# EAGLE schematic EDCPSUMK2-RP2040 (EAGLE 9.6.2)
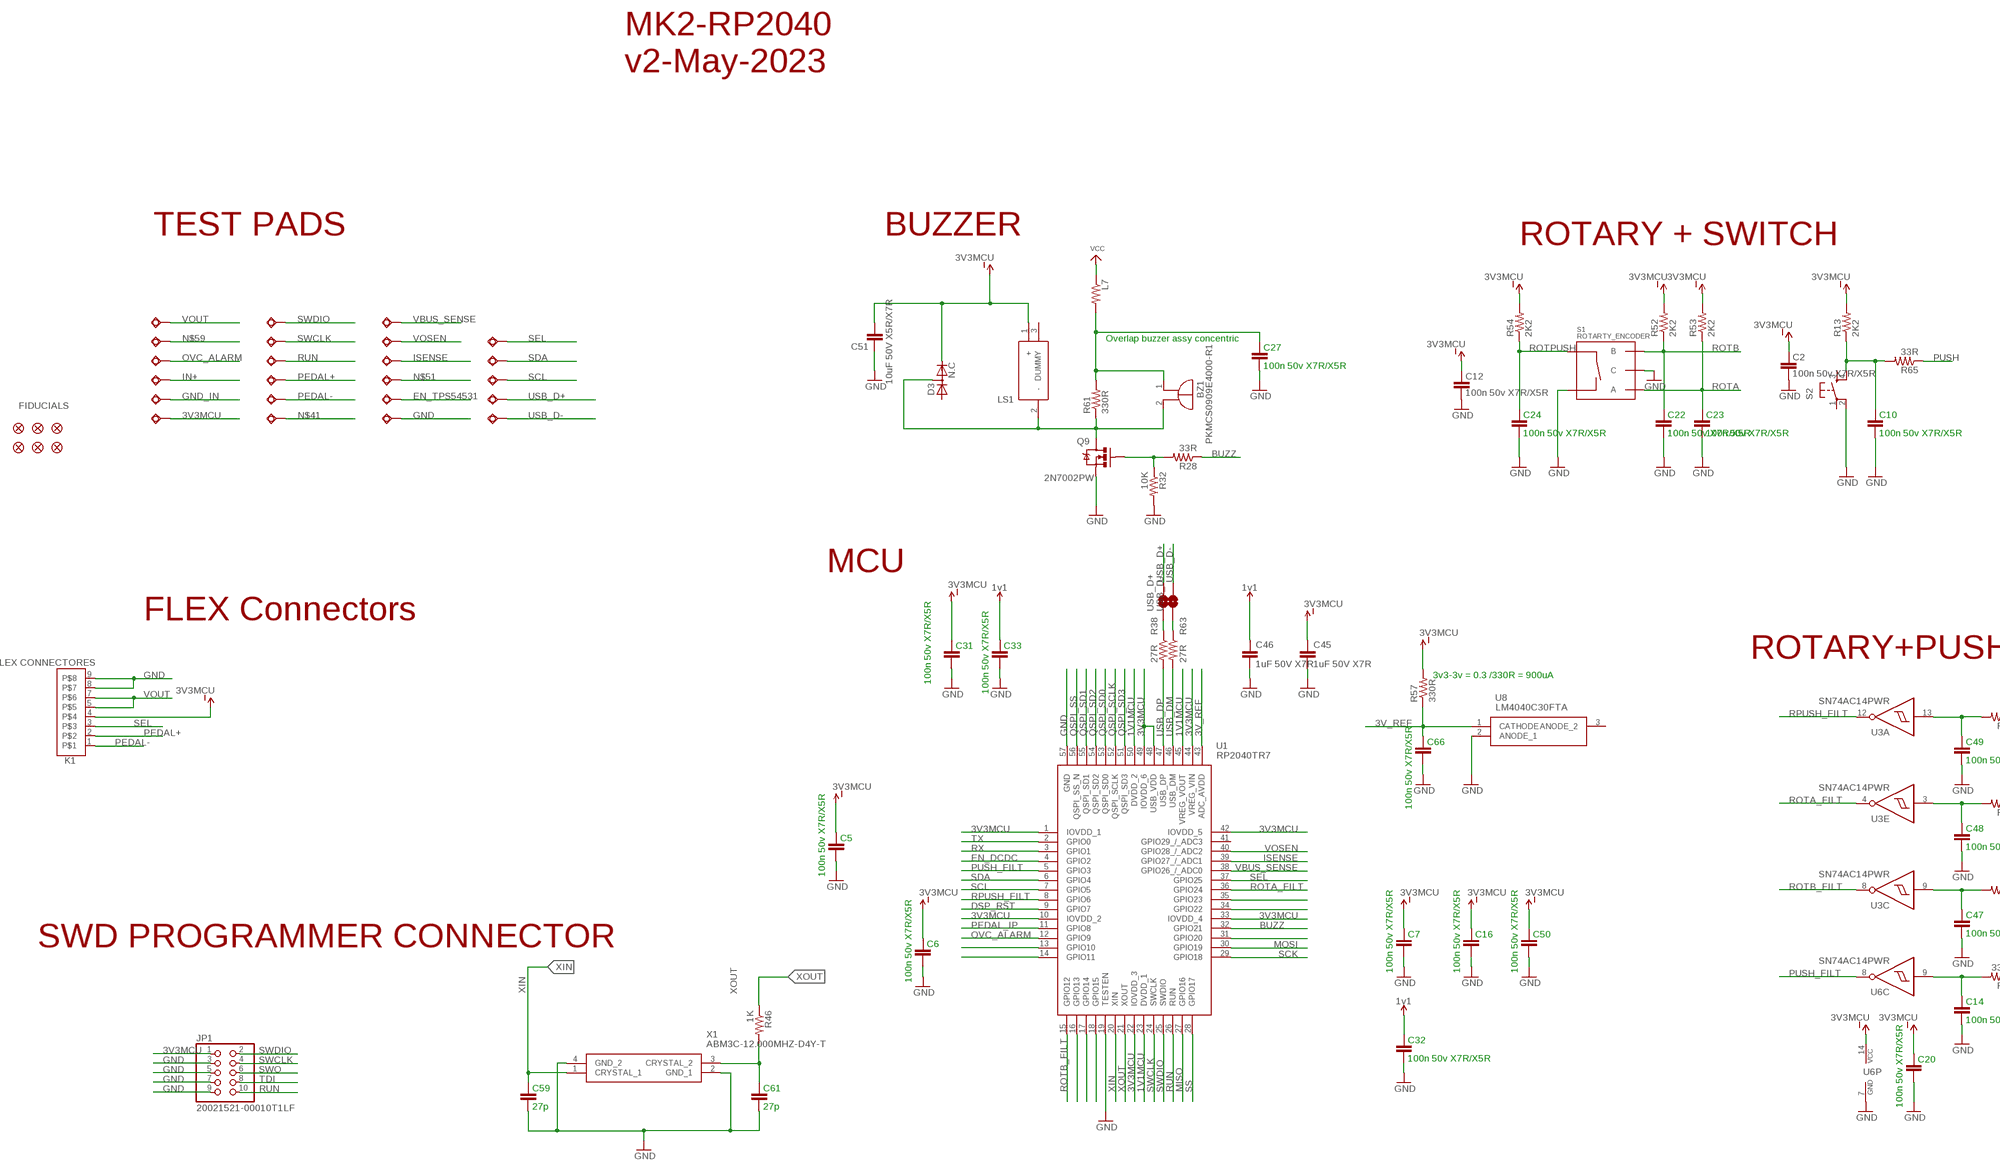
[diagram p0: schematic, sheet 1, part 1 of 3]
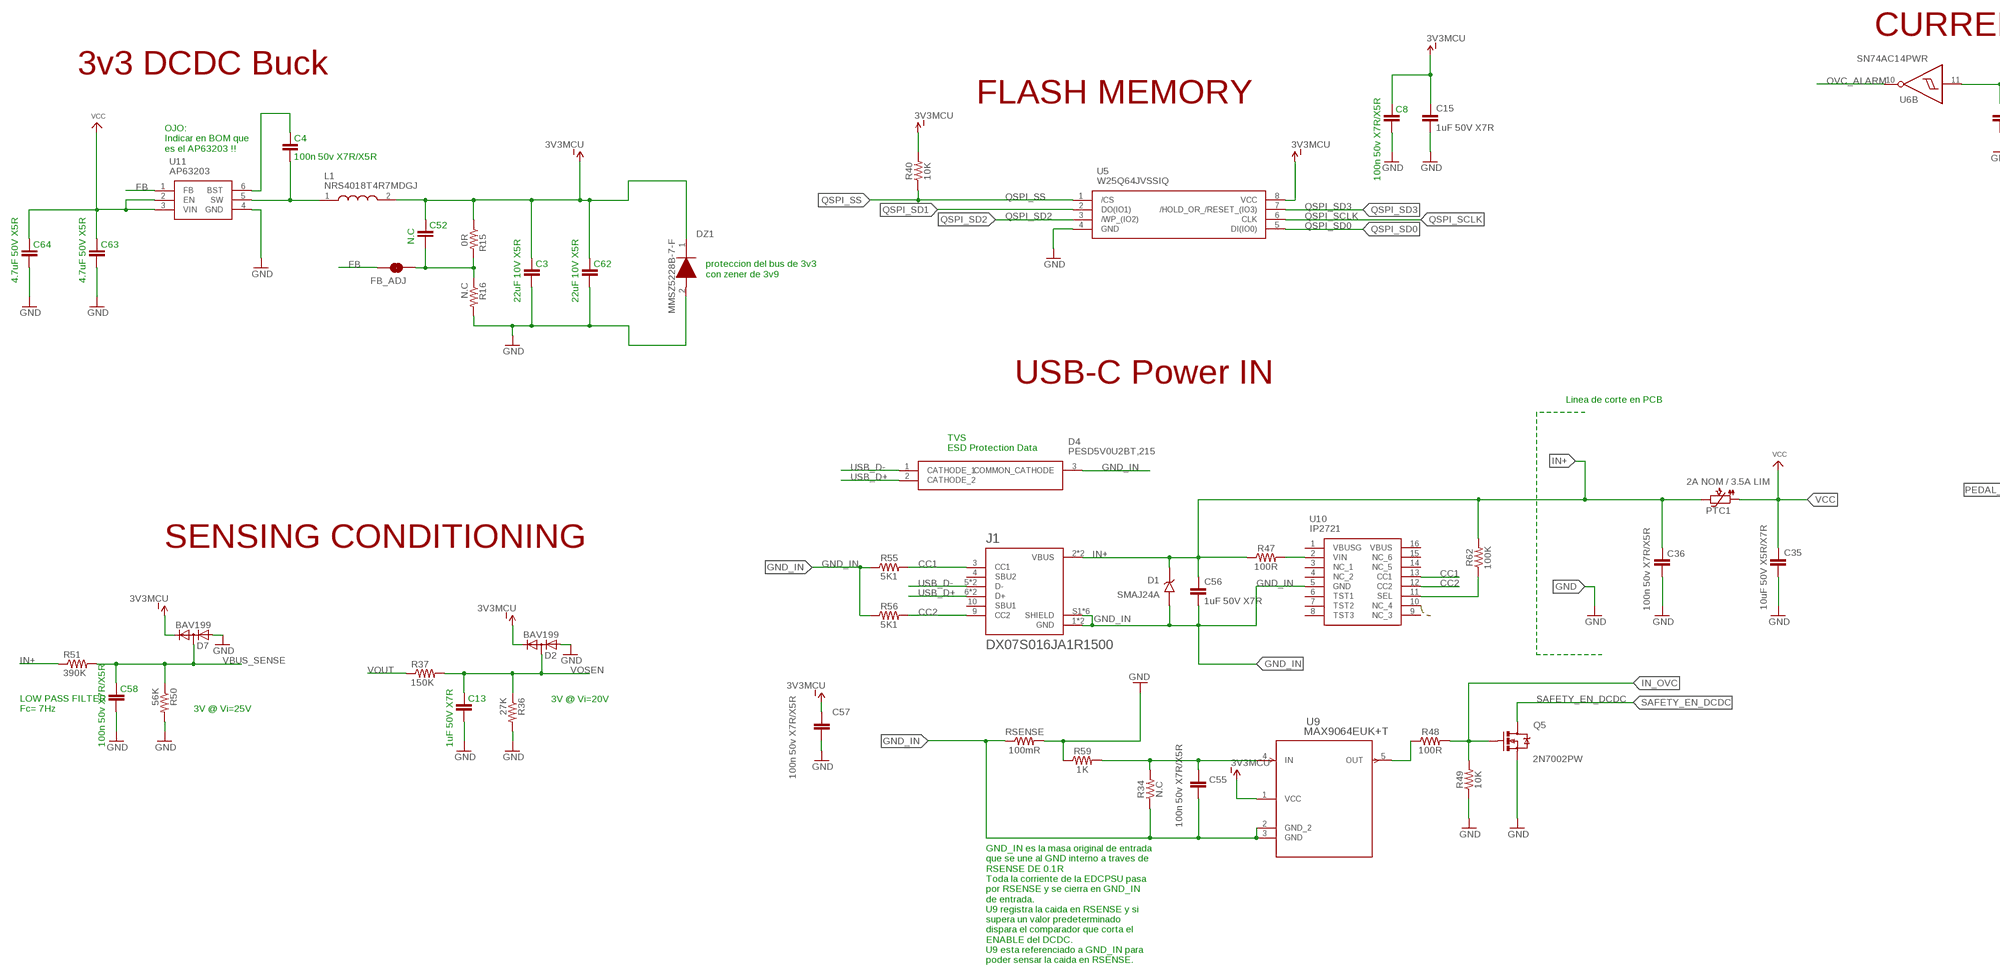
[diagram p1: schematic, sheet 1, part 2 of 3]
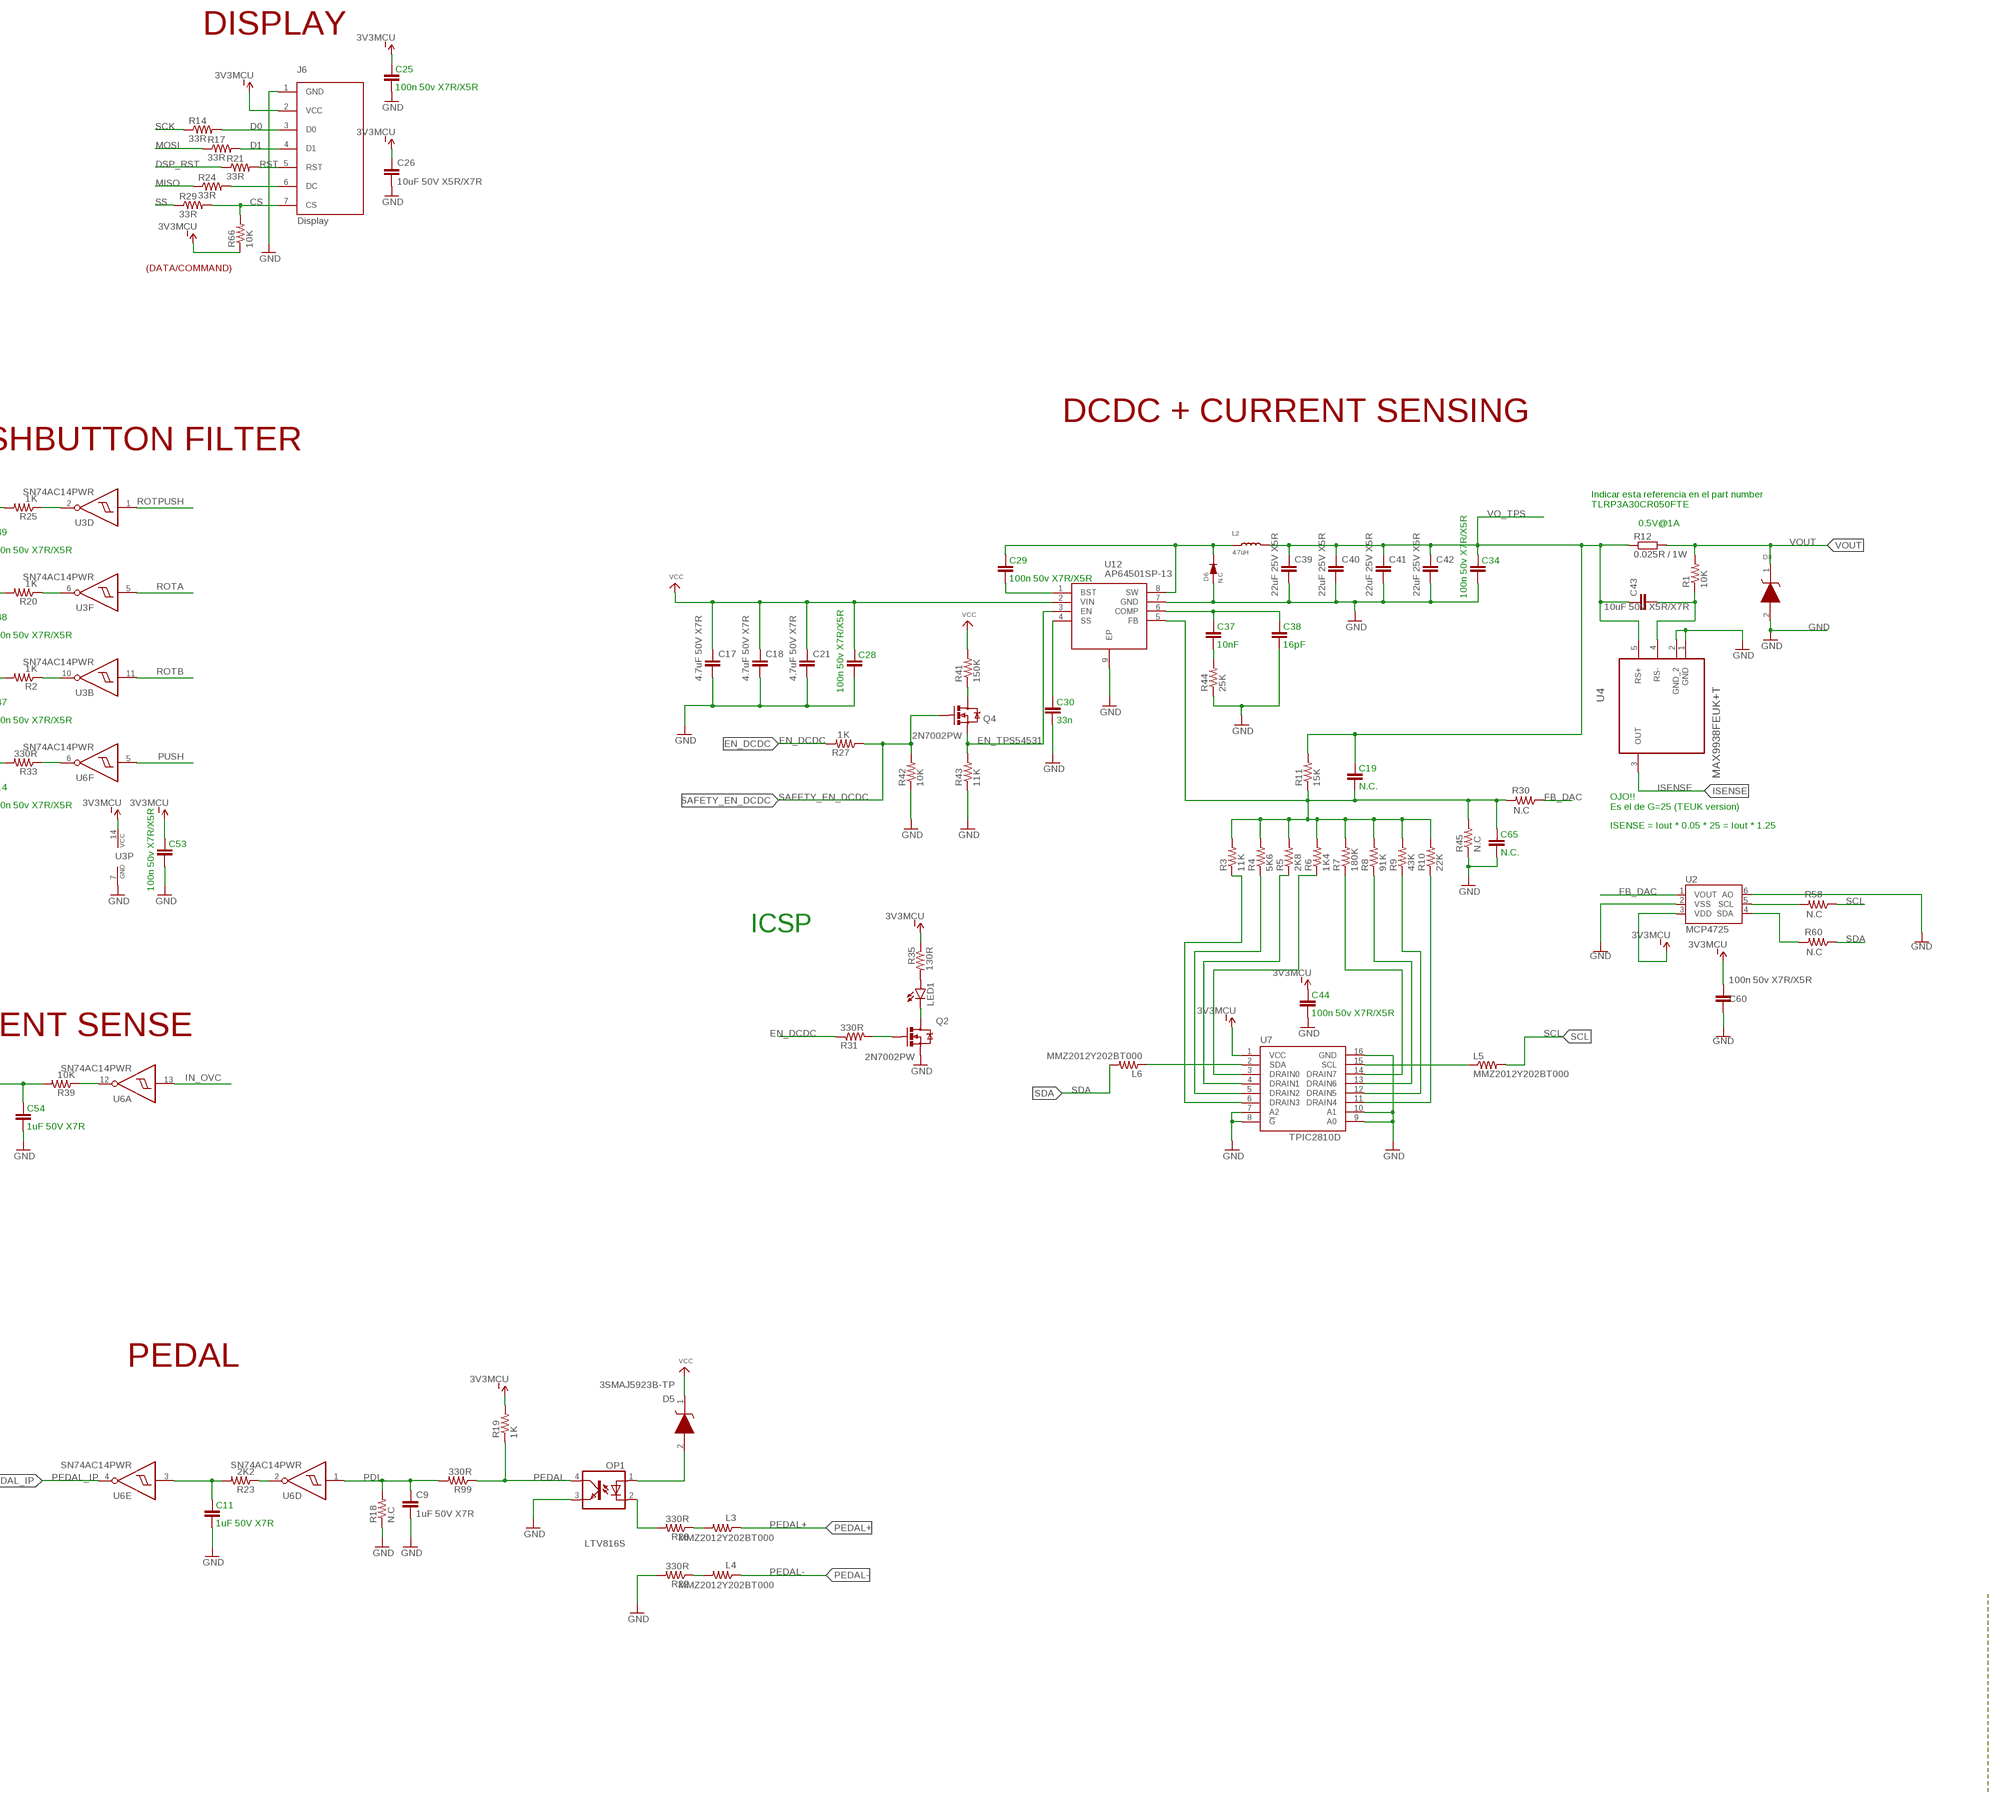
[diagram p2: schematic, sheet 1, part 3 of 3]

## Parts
3V3MCU  TESTPAD_TPSQB1,27  [TESTPAD_B1,27]
BZ1  PKMCS0909E4000-R1  [PKMCS0909]
C2  100n 50v X7R/X5R  CAP0805  [0805]
C3  22uF 10V X5R  CAP0805  [0805]
C4  100n 50v X7R/X5R  CAP0805  [0805]
C5  100n 50v X7R/X5R  CAP0805  [0805]
C6  100n 50v X7R/X5R  CAP0805  [0805]
C7  100n 50v X7R/X5R  CAP0805  [0805]
C8  100n 50v X7R/X5R  CAP0805  [0805]
C9  1uF 50V X7R  CAP0805  [0805]
C10  100n 50v X7R/X5R  CAP0805  [0805]
C11  1uF 50V X7R  CAP0805  [0805]
C12  100n 50v X7R/X5R  CAP0805  [0805]
C13  1uF 50V X7R  CAP0805  [0805]
C14  100n 50v X7R/X5R  CAP0805  [0805]
C15  1uF 50V X7R  CAP0805  [0805]
C16  100n 50v X7R/X5R  CAP0805  [0805]
C17  4.7uF 50V X7R  CAP1210  [1210]
C18  4.7uF 50V X7R  CAP1210  [1210]
C19  N.C.  CAP0805  [0805]
C20  100n 50v X7R/X5R  CAP0805  [0805]
C21  4.7uF 50V X7R  CAP1210  [1210]
C22  100n 50v X7R/X5R  CAP0805  [0805]
C23  100n 50v X7R/X5R  CAP0805  [0805]
C24  100n 50v X7R/X5R  CAP0805  [0805]
C25  100n 50v X7R/X5R  CAP0805  [0805]
C26  10uF 50V X5R/X7R  CAP1206  [1206]
C27  100n 50v X7R/X5R  CAP0805  [0805]
C28  100n 50v X7R/X5R  CAP0805  [0805]
C29  100n 50v X7R/X5R  CAP0805  [0805]
C30  33n  CAP0805  [0805]
C31  100n 50v X7R/X5R  CAP0805  [0805]
C32  100n 50v X7R/X5R  CAP0805  [0805]
C33  100n 50v X7R/X5R  CAP0805  [0805]
C34  100n 50v X7R/X5R  CAP0805  [0805]
C35  10uF 50V X5R/X7R  CAP1206  [1206]
C36  100n 50v X7R/X5R  CAP0805  [0805]
C37  10nF  CAP0805  [0805]
C38  16pF  CAP0805  [0805]
C39  22uF 25V X5R  CAP1210  [1210]
C40  22uF 25V X5R  CAP1210  [1210]
C41  22uF 25V X5R  CAP1210  [1210]
C42  22uF 25V X5R  CAP1210  [1210]
C43  10uF 50V X5R/X7R  CAP1206  [1206]
C44  100n 50v X7R/X5R  CAP0805  [0805]
C45  1uF 50V X7R  CAP0805  [0805]
C46  1uF 50V X7R  CAP0805  [0805]
C47  100n 50v X7R/X5R  CAP0805  [0805]
C48  100n 50v X7R/X5R  CAP0805  [0805]
C49  100n 50v X7R/X5R  CAP0805  [0805]
C50  100n 50v X7R/X5R  CAP0805  [0805]
C51  10uF 50V X5R/X7R  CAP1206  [1206]
C52  N.C  CAP0805  [0805]
C53  100n 50v X7R/X5R  CAP0805  [0805]
C54  1uF 50V X7R  CAP0805  [0805]
C55  100n 50v X7R/X5R  CAP0805  [0805]
C56  1uF 50V X7R  CAP0805  [0805]
C57  100n 50v X7R/X5R  CAP0805  [0805]
C58  100n 50v X7R/X5R  CAP0805  [0805]
C59  27p  CAP0805  [0805]
C60  100n 50v X7R/X5R  CAP0805  [0805]
C61  27p  CAP0805  [0805]
C62  22uF 10V X5R  CAP0805  [0805]
C63  4.7uF 50V X5R  CAP0805  [0805]
C64  4.7uF 50V X5R  CAP0805  [0805]
C65  N.C.  CAP0805  [0805]
C66  100n 50v X7R/X5R  CAP0805  [0805]
D1  SMAJ24A  3SMAJ5934B  [DIOM4325X244N]
D2  BAV199  [SOT23]
D3  N.C  BAV199  [SOT23]
D4  PESD5V0U2BT,215  [SOT95P230X110-3N]
D5  3SMAJ5923B-TP  [DIOM5226X244N]
D6  N.C  DSMC  [DO-214AB]
D7  BAV199  [SOT23]
D8  RB060M-60TR  3SMAJ5923B-TP  [DIOM5226X244N]
DZ1  MMSZ5228B-7-F  [SODFL3518X115N]
EN_TPS54531  TESTPAD_TPSQB1,27  [TESTPAD_B1,27]
FB_ADJ  JUMPER-SMT_2_NC_TRACE_NO-SILK  [SMT-JUMPER_2_NC_TRACE_NO-SILK]
FID1  FIDUCIAL1X2  [FIDUCIAL-1X2]
FID2  FIDUCIAL1X2  [FIDUCIAL-1X2]
FID3  FIDUCIAL1X2  [FIDUCIAL-1X2]
FID4  FIDUCIAL1X2  [FIDUCIAL-1X2]
FID5  FIDUCIAL1X2  [FIDUCIAL-1X2]
FID6  FIDUCIAL1X2  [FIDUCIAL-1X2]
GND  TESTPAD_TPSQB1,27  [TESTPAD_B1,27]
GND_IN  TESTPAD_TPSQB1,27  [TESTPAD_B1,27]
IN+  TESTPAD_TPSQB1,27  [TESTPAD_B1,27]
ISENSE  TESTPAD_TPSQB1,27  [TESTPAD_B1,27]
J1  DX07S016JA1R1500  [JAE_DX07S016JA1R1500]
J6  Display  OLED_LCD  [OLED_LCD]
JP1  20021521-00010T1LF  [20021521-00010T1LF]
K1  FLEX CONNECTORES  FLEX8  [FLEX8]
L1  NRS4018T4R7MDGJ  [NRS4018T100MDGJ]
L2  4.7uH  L74437368047  [WE-LHMI]
L3  MMZ2012Y202BT000  RESISTOR0805-RES  [0805]
L4  MMZ2012Y202BT000  RESISTOR0805-RES  [0805]
L5  MMZ2012Y202BT000  RESISTOR0805-RES  [0805]
L6  MMZ2012Y202BT000  RESISTOR0805-RES  [0805]
L7  MMZ2012Y202BT000  RESISTOR0805-RES  [0805]
LED1  LED3MM  [LED3MM]
LS1  SMT-0540-S-R  [SMT0540SR]
N$41  TESTPAD_TPSQB1,27  [TESTPAD_B1,27]
N$51  TESTPAD_TPSQB1,27  [TESTPAD_B1,27]
N$59  TESTPAD_TPSQB1,27  [TESTPAD_B1,27]
OP1  LTV816S  [SMD4]
OVC_ALARM  TESTPAD_TPSQB1,27  [TESTPAD_B1,27]
PEDAL+  TESTPAD_TPSQB1,27  [TESTPAD_B1,27]
PEDAL-  TESTPAD_TPSQB1,27  [TESTPAD_B1,27]
PTC1  2A NOM / 3.5A LIM  PTC-  [1812L]
Q2  2N7002PW  MOSFET-NCHANNEL2N7002PW  [SOT323]
Q4  2N7002PW  MOSFET-NCHANNEL2N7002PW  [SOT323]
Q5  2N7002PW  MOSFET-NCHANNEL2N7002PW  [SOT323]
Q9  2N7002PW  MOSFET-NCHANNEL2N7002PW  [SOT323]
R1  10K  RESISTOR0805  [0805]
R2  1K  RESISTOR0805  [0805]
R3  11K  RESISTOR0805  [0805]
R4  5K6  RESISTOR0805  [0805]
R5  2K8  RESISTOR0805  [0805]
R6  1K4  RESISTOR0805  [0805]
R7  180K  RESISTOR0805  [0805]
R8  91K  RESISTOR0805  [0805]
R9  43K  RESISTOR0805  [0805]
R10  22K  RESISTOR0805  [0805]
R11  15K  RESISTOR0805  [0805]
R12  0.025R / 1W  RR2512  [R2512]
R13  2K2  RESISTOR0805  [0805]
R14  33R  RESISTOR0805  [0805]
R15  0R  RESISTOR0805  [0805]
R16  N.C  RESISTOR0805  [0805]
R17  33R  RESISTOR0805  [0805]
R18  N.C  RESISTOR0805  [0805]
R19  1K  RESISTOR0805  [0805]
R20  1K  RESISTOR0805  [0805]
R21  33R  RESISTOR0805  [0805]
R22  330R  RESISTOR0805  [0805]
R23  2K2  RESISTOR0805  [0805]
R24  33R  RESISTOR0805  [0805]
R25  1K  RESISTOR0805  [0805]
R26  330R  RESISTOR0805  [0805]
R27  1K  RESISTOR0805  [0805]
R28  33R  RESISTOR0805  [0805]
R29  33R  RESISTOR0805  [0805]
R30  N.C  RESISTOR0805  [0805]
R31  330R  RESISTOR0805  [0805]
R32  10K  RESISTOR0805  [0805]
R33  330R  RESISTOR0805  [0805]
R34  N.C  RESISTOR0805  [0805]
R35  130R  RESISTOR0805  [0805]
R36  27K  RESISTOR0805  [0805]
R37  150K  RESISTOR0805  [0805]
R38  27R  RESISTOR0805  [0805]
R39  10K  RESISTOR0805  [0805]
R40  10K  RESISTOR0805  [0805]
R41  150K  RESISTOR0805  [0805]
R42  10K  RESISTOR0805  [0805]
R43  11K  RESISTOR0805  [0805]
R44  25K  RESISTOR0805  [0805]
R45  N.C  RESISTOR0805  [0805]
R46  1K  RESISTOR0805  [0805]
R47  100R  RESISTOR0805  [0805]
R48  100R  RESISTOR0805  [0805]
R49  10K  RESISTOR0805  [0805]
R50  56K  RESISTOR0805  [0805]
R51  390K  RESISTOR0805  [0805]
R52  2K2  RESISTOR0805  [0805]
R53  2K2  RESISTOR0805  [0805]
R54  2K2  RESISTOR0805  [0805]
R55  5K1  RESISTOR0805  [0805]
R56  5K1  RESISTOR0805  [0805]
R57  330R  RESISTOR0805  [0805]
R58  N.C  RESISTOR0805  [0805]
R59  1K  RESISTOR0805  [0805]
R60  N.C  RESISTOR0805  [0805]
R61  330R  RESISTOR0805  [0805]
R62  100K  RESISTOR0805  [0805]
R63  27R  RESISTOR0805  [0805]
R65  33R  RESISTOR0805  [0805]
R66  10K  RESISTOR0805  [0805]
R99  330R  RESISTOR0805  [0805]
RSENSE  100mR  RESISTOR1206  [1206]
RUN  TESTPAD_TPSQB1,27  [TESTPAD_B1,27]
S1  ROTARTY_ENCODER  [ROTARY_ENC_PLAIN]
S2  TAC_SWITCH_KSC931G-SMD  [TAC_SW_SMD_KSC931G]
SCL  TESTPAD_TPSQB1,27  [TESTPAD_B1,27]
SDA  TESTPAD_TPSQB1,27  [TESTPAD_B1,27]
SEL  TESTPAD_TPSQB1,27  [TESTPAD_B1,27]
SWCLK  TESTPAD_TPSQB1,27  [TESTPAD_B1,27]
SWDIO  TESTPAD_TPSQB1,27  [TESTPAD_B1,27]
U1  RP2040TR7  [RP2040TR7]
U2  MCP4725  MCP4725SOT-23  [SOT23-6]
U3  SN74AC14PWR  7414  [TSSOP14]
U4  MAX9938FEUK+T  [SOT95P280X145-5N]
U5  W25Q64JVSSIQ  [SOIC127P790X216-8N]
U6  SN74AC14PWR  7414  [TSSOP14]
U7  TPIC2810D  [SO16]
U8  LM4040C30FTA  [SOT96P240X120-3N]
U9  MAX9064EUK+T  [21-0057F_MXM]
U10  IP2721  [SOP65P640X120-16N]
U11  AP63203  AP63201WU-7  [SOT95P280X100-6N]
U12  AP64501SP-13  [SOIC127P600X163-9N]
USB-D+  TESTPAD_TPSQB1,27  [TESTPAD_B1,27]
USB-D-  TESTPAD_TPSQB1,27  [TESTPAD_B1,27]
USB_D+  JUMPER-SMT_2_NO_NO-SILK  [SMT-JUMPER_2_NO_NO-SILK]
USB_D-  JUMPER-SMT_2_NO_NO-SILK  [SMT-JUMPER_2_NO_NO-SILK]
VBUS_SENSE  TESTPAD_TPSQB1,27  [TESTPAD_B1,27]
VOSEN  TESTPAD_TPSQB1,27  [TESTPAD_B1,27]
VOUT  TESTPAD_TPSQB1,27  [TESTPAD_B1,27]
X1  ABM3C-12.000MHZ-D4Y-T  [ABM3C16000MHZD4YT]

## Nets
1V1MCU: C32.2 C33.2 C46.1 U1.23(DVDD_1) U1.45(VREG_VOUT) U1.50(DVDD_2) ; supply symbol labelled 1v1
3V3MCU: 3V3MCU.TP C2.2 C3.2 C5.2 C6.2 C7.2 C8.2 C12.2 C15.1 C16.2 C20.2 C25.2 C26.1 C31.2 C44.2 C45.1 C50.2 C51.2 C52.2 C53.2 C57.1 C60.2 C62.2 D2.2(C) D3.2(C) D7.2(C) DZ1.1(K) J6.2(VCC) JP1.1 K1.4 L1.2 LS1.1(+) R13.2 R15.1 R19.2 R35.1 R40.2 R52.2 R53.2 R54.2 R57.2 R66.1 U1.1(IOVDD_1) U1.10(IOVDD_2) U1.22(IOVDD_3) U1.33(IOVDD_4) U1.42(IOVDD_5) U1.44(VREG_VIN) U1.48(USB_VDD) U1.49(IOVDD_6) U2.3(VDD) U3.14(P:VCC) U5.8(VCC) U6.14(P:VCC) U7.1(VCC) U9.1(VCC)
3V_REF: C66.2 R57.1 U1.43(ADC_AVDD) U8.1(CATHODE)
BUZZ: R28.1 U1.32(GPIO21)
CC1: J1.3(CC1) R55.2 U10.13(CC1)
CC2: J1.9(CC2) R56.2 U10.12(CC2)
CS: J6.7(CS) R29.2 R66.2
D0: J6.3(D0) R14.2
D1: J6.4(D1) R17.2
DSP_RST: R21.1 U1.9(GPIO7)
EN_DCDC: R27.2 R31.1 U1.4(GPIO2)
EN_TPS54531: EN_TPS54531.TP Q4.2(S) R43.2 U12.3(EN)
FB: FB_ADJ.2 U11.1(FB)
FB_DAC: R30.1 U2.1(VOUT)
GND: C2.1 C3.1 C5.1 C6.1 C7.1 C8.1 C9.2 C10.1 C11.1 C12.1 C13.1 C14.1 C15.2 C16.1 C17.2 C18.2 C20.1 C21.2 C22.1 C23.1 C24.1 C25.1 C26.2 C27.1 C28.1 C30.1 C31.1 C32.1 C33.1 C34.1 C35.2 C36.1 C38.1 C39.2 C40.2 C41.2 C42.2 C44.1 C45.2 C46.2 C47.1 C48.1 C49.1 C50.1 C51.1 C53.1 C54.1 C57.2 C58.1 C59.1 C60.1 C61.1 C62.1 C63.1 C64.1 C65.1 C66.1 D2.1(A) D6.1(A) D7.1(A) D8.2(A) DZ1.2(A) GND.TP J6.1(GND) JP1.3 JP1.5 JP1.7 JP1.9 K1.8 K1.9 OP1.3(EMIT) Q2.2(S) Q5.2(S) Q9.2(S) R16.2 R18.1 R22.2 R32.2 R36.2 R42.1 R43.1 R44.1 R45.1 R49.1 R50.2 R59.1 RSENSE.2 S1.C S1.SW- S2.2 U1.19(TESTEN) U1.57(GND) U2.2(VSS) U2.6(AO) U3.7(P:GND) U4.1(GND) U4.2(GND_2) U5.4(GND) U6.7(P:GND) U7.7(A2) U7.8(!G) U7.9(A0) U7.10(A1) U7.16(GND) U8.2(ANODE_1) U11.4(GND) U12.7(GND) U12.9(EP) X1.2(GND_1) X1.4(GND_2)
GND_IN: C55.2 C56.2 D1.A D4.3(COMMON_CATHODE) GND_IN.TP J1.1(GND) J1.12(GND) J1.S1(SHIELD) J1.S2(SHIELD) J1.S3(SHIELD) J1.S4(SHIELD) J1.S5(SHIELD) J1.S6(SHIELD) R34.1 R55.1 R56.1 RSENSE.1 U9.2(GND_2) U9.3(GND) U10.5(GND)
IN+: C36.2 C56.1 D1.C(K) IN+.TP J1.2(VBUS) J1.11(VBUS) PTC1.2 R47.1 R51.1 R62.2
IN_OVC: Q5.1(G) R48.2 R49.2 U6.13(A:I)
ISENSE: ISENSE.TP U1.39(GPIO27_/_ADC1) U4.3(OUT)
MISO: R24.1 U1.27(GPIO16)
MOSI: R17.1 U1.30(GPIO19)
N$1: R3.1 U7.6(DRAIN3)
N$2: R4.1 U7.5(DRAIN2)
N$3: R5.1 U7.4(DRAIN1)
N$4: R6.1 U7.3(DRAIN0)
N$5: R7.1 U7.14(DRAIN7)
N$6: J6.6(DC) R24.2
N$7: R8.1 U7.13(DRAIN6)
N$8: R9.1 U7.12(DRAIN5)
N$9: R10.1 U7.11(DRAIN4)
N$10: C43.2 R1.1 U4.4(RS-)
N$11: LED1.A R35.2
N$12: LED1.K(C) Q2.3(D)
N$13: R33.1 U6.6(F:O)
N$14: R62.1 U10.11(SEL)
N$15: R39.1 U6.12(A:O)
N$16: D5.2(A) OP1.1(A)
N$17: C10.2 R13.1 R65.2 S2.4
N$18: C47.2 R2.2 U3.9(C:I)
N$19: C19.1 C65.2 R3.2 R4.2 R5.2 R6.2 R7.2 R8.2 R9.2 R10.2 R11.1 R30.2 R45.2 U12.5(FB)
N$20: Q9.1(G) R28.2 R32.1
N$21: Q2.1(G) R31.2
N$22: R2.1 U3.10(B:O)
N$23: R20.1 U3.6(F:O)
N$25: R25.1 U3.2(D:O)
N$26: C49.2 R25.2 U3.13(A:I)
N$28: C48.2 R20.2 U3.3(E:I)
N$29: C11.2 R23.2 U6.3(E:I)
N$31: BZ1.2(-) D3.3(AC) LS1.2(-) Q9.3(D) R61.1
N$32: BZ1.1(+) C27.2 L7.2 R61.2
N$34: R23.1 U6.2(D:O)
N$35: Q4.3(D) R41.1
N$37: C14.2 R33.2 U6.9(C:I)
N$38: C52.1 FB_ADJ.1 R15.2 R16.1
N$39: C54.2 R39.2 U6.11(B:I)
N$40: L6.1 U7.2(SDA)
N$41: N$41.TP OP1.2(C) R26.2
N$43: L3.2 R26.1
N$44: C30.2 U12.4(SS)
N$45: R58.2 U2.5(SCL)
N$46: L4.2 R22.1
N$47: C29.1 U12.1(BST)
N$48: R60.2 U2.4(SDA)
N$49: U1.35(GPIO23)
N$50: R47.2 U10.2(VIN)
N$51: C29.2 D6.2(K) L2.1 N$51.TP U12.8(SW)
N$52: C37.2 C38.2 U12.6(COMP)
N$53: C37.1 R44.2
N$54: L5.1 U7.15(SCL)
N$55: U1.34(GPIO22)
N$56: C4.2 U11.6(BST)
N$58: R48.1 U9.5(OUT)
N$59: C55.1 N$59.TP R34.2 R59.2 U9.4(IN)
N$60: U1.31(GPIO20)
N$63: C61.2 R46.2 X1.3(CRYSTAL_2)
N$64: R38.1 USB_D+.1
N$65: R63.1 USB_D-.1
N$67: C4.1 L1.1 U11.5(SW)
N$82: U1.13(GPIO10)
N$83: U1.14(GPIO11)
N$85: U1.16(GPIO13)
N$86: U1.17(GPIO14)
N$87: U1.18(GPIO15)
OVC_ALARM: OVC_ALARM.TP U1.12(GPIO9) U6.10(B:O)
PDL: C9.1 R18.2 R99.2 U6.1(D:I)
PEDAL: OP1.4(COL) R19.1 R99.1
PEDAL+: K1.2 L3.1 PEDAL+.TP
PEDAL-: K1.1 L4.1 PEDAL-.TP
PEDAL_IP: U1.11(GPIO8) U6.4(E:O)
PUSH: R65.1 U6.5(F:I)
PUSH_FILT: U1.5(GPIO3) U6.8(C:O)
QSPI_SCLK: U1.52(QSPI_SCLK) U5.6(CLK)
QSPI_SD0: U1.53(QSPI_SD0) U5.5(DI(IO0))
QSPI_SD1: U1.55(QSPI_SD1) U5.2(DO(IO1))
QSPI_SD2: U1.54(QSPI_SD2) U5.3(/WP_(IO2))
QSPI_SD3: U1.51(QSPI_SD3) U5.7(/HOLD_OR_/RESET_(IO3))
QSPI_SS: R40.1 U1.56(QSPI_SS_N) U5.1(/CS)
ROTA: C23.2 R53.1 S1.A U3.5(F:I)
ROTA_FILT: U1.36(GPIO24) U3.4(E:O)
ROTB: C22.2 R52.1 S1.B U3.11(B:I)
ROTB_FILT: U1.15(GPIO12) U3.8(C:O)
ROTPUSH: C24.2 R54.1 S1.SW+ U3.1(D:I)
RPUSH_FILT: U1.8(GPIO6) U3.12(A:O)
RST: J6.5(RST) R21.2
RUN: JP1.10 RUN.TP U1.26(RUN)
RX: U1.3(GPIO1)
SAFETY_EN_DCDC: Q4.1(G) Q5.3(D) R27.1 R42.2
SCK: R14.1 U1.29(GPIO18)
SCL: L5.2 R58.1 SCL.TP U1.7(GPIO5)
SDA: L6.2 R60.1 SDA.TP U1.6(GPIO4)
SEL: K1.3 SEL.TP U1.37(GPIO25)
SS: R29.1 U1.28(GPIO17)
SWCLK: JP1.4 SWCLK.TP U1.24(SWCLK)
SWDIO: JP1.2 SWDIO.TP U1.25(SWDIO)
SWO: JP1.6
TDI: JP1.8
TX: U1.2(GPIO0)
USB_D+: D4.2(CATHODE_2) J1.6(D+) J1.7(D+) USB-D+.TP USB_D+.2
USB_D-: D4.1(CATHODE_1) J1.5(D-) J1.8(D-) USB-D-.TP USB_D-.2
USB_DM: R63.2 U1.46(USB_DM)
USB_DP: R38.2 U1.47(USB_DP)
VBUS_SENSE: C58.2 D7.3(AC) R50.1 R51.2 U1.38(GPIO26_/_ADC0) VBUS_SENSE.TP
VCC: C17.1 C18.1 C21.1 C28.2 C35.1 C63.2 C64.2 D5.1(K) L7.1 PTC1.1 R41.2 U11.2(EN) U11.3(VIN) U12.2(VIN)
VO_TPS: C19.2 C34.2 C39.1 C40.1 C41.1 C42.1 C43.1 L2.2 R11.2 R12.1 U4.5(RS+)
VOSEN: C13.2 D2.3(AC) R36.1 R37.2 U1.40(GPIO28_/_ADC2) VOSEN.TP
VOUT: D8.1(K) K1.5 K1.7 R1.2 R12.2 R37.1 VOUT.TP
XIN: C59.2 U1.20(XIN) X1.1(CRYSTAL_1)
XOUT: R46.1 U1.21(XOUT)
Unconnected: D3.1(A) J1.4(SBU2) J1.10(SBU1) LS1.3(DUMMY) S2.1 S2.3 U1.41(GPIO29_/_ADC3) U8.3(ANODE_2) U10.1(VBUSG) U10.3(NC_1) U10.4(NC_2) U10.6(TST1) U10.7(TST2) U10.8(TST3) U10.9(NC_3) U10.10(NC_4) U10.14(NC_5) U10.15(NC_6) U10.16(VBUS)

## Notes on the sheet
- MK2-RP2040
  v2-May-2023
- TEST PADS | BUZZER | ROTARY + SWITCH | DISPLAY
- Overlap buzzer assy concentric
- FIDUCIALS
- (DATA/COMMAND)
- MCU
- FLEX Connectors | DCDC + CURRENT SENSING
- ROTARY+PUSHBUTTON FILTER
- 3v3-3v = 0.3 /330R = 900uA
- Indicar esta referencia en el part number
  TLRP3A30CR050FTE
- 0.5V@1A
- SWD PROGRAMMER CONNECTOR
- OJO!!
  Es el de G=25 (TEUK version)
- ISENSE = Iout * 0.05 * 25 = Iout * 1.25
- ICSP
- CURRENT SENSE
- 3v3 DCDC Buck
- FLASH MEMORY
- OJO:
  Indicar en BOM que 
  es el AP63203 !!
- proteccion del bus de 3v3
  con zener de 3v9
- USB-C Power IN | PEDAL
- Linea de corte en PCB
- TVS
  ESD Protection Data
- SENSING CONDITIONING
- 3V @ Vi=20V
- LOW PASS FILTER
  Fc= 7Hz
- 3V @ Vi=25V
- GND_IN es la masa original de entrada
  que se une al GND interno a traves de
  RSENSE DE 0.1R
  Toda la corriente de la EDCPSU pasa 
  por RSENSE y se cierra en GND_IN
  de entrada.
  U9 registra la caida en RSENSE y si
  supera un valor predeterminado
  dispara el comparador que corta el 
  ENABLE del DCDC.
  U9 esta referenciado a GND_IN para
  poder sensar la caida en RSENSE.

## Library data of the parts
3V3MCU EN_TPS54531 GND GND_IN IN+ ISENSE N$41 N$51 N$59 OVC_ALARM PEDAL+ PEDAL- RUN SCL SDA SEL SWCLK SWDIO USB-D+ USB-D- VBUS_SENSE VOSEN VOUT = BeagleBone_Blue_R3:TESTPAD_TPSQ: Test pad
BZ1 = buzzer:PKMCS0909E4000-R1: PKMCS0909E4000-R1
C2-C66 = SparkFun-Passives:CAP: Capacitor
D1 = 3SMAJ5934B:3SMAJ5934B: Check availability; AVAILABILITY: Not in stock; DESCRIPTION: Zener Diode Single 24V 5% 19Ohm 3000mW 2-Pin SMA T/R; MF: Micro Commercial Components; MP: 3SMAJ5934B; PACKAGE: None; PRICE: None
D2 D3 D7 = diode:BAV199: DIODE low-leakage double diode
D4 = PESD5V0U2BT_215:PESD5V0U2BT,215: PESD5V0U2BT - Ultra low capacitance bidirectional double ESD protection diode Source: Datasheet; ARROW_PART_NUMBER: PESD5V0U2BT,215; ARROW_PRICE-STOCK: https://www.arrow.com/en/products/pesd5v0u2bt215/nexperia?region=nac; DESCRIPTION: PESD5V0U2BT - Ultra low capacitance bidirectional double ESD protection diode; HEIGHT: 1.1mm; MANUFACTURER_NAME: Nexperia; MANUFACTURER_PART_NUMBER: PESD5V0U2BT,215; MOUSER_PART_NUMBER: 771-PESD5V0U2BTT/R; MOUSER_PRICE-STOCK: https://www.mouser.co.uk/ProductDetail/Nexperia/PESD5V0U2BT215?qs=LOCUfHb8d9uKnndgcTorSw%3D%3D
D5 D8 = 3SMAJ5923B-TP:3SMAJ5923B-TP: Zener Diodes 3W 8.2V; ARROW_PART_NUMBER: 3SMAJ5923B-TP; ARROW_PRICE-STOCK: https://www.arrow.com/en/products/3smaj5923b-tp/micro-commercial-components; DESCRIPTION: Zener Diodes 3W 8.2V; HEIGHT: 2.44mm; MANUFACTURER_NAME: MCC; MANUFACTURER_PART_NUMBER: 3SMAJ5923B-TP; MOUSER_PART_NUMBER: 833-3SMAJ5923B-TP; MOUSER_PRICE-STOCK: https://www.mouser.com/Search/Refine.aspx?Keyword=833-3SMAJ5923B-TP
D6 = EDCPSU - Rev3:D*
DZ1 = MMSZ5228B-7-F:MMSZ5228B-7-F: Diodes Inc MMSZ5228B-7-F Zener Diode, 3.9V 5% 500 mW SMT 2-Pin SOD-123; DESCRIPTION: Diodes Inc MMSZ5228B-7-F Zener Diode, 3.9V 5% 500 mW SMT 2-Pin SOD-123; HEIGHT: 1.15mm; MANUFACTURER_NAME: Diodes Inc.; MANUFACTURER_PART_NUMBER: MMSZ5228B-7-F
FB_ADJ = SparkFun-Jumpers:JUMPER-SMT_2_NC_TRACE: Normally closed trace jumper
FID1-FID6 = SparkFun-Aesthetics:FIDUCIAL: Fiducial Alignment Points
J1 = DX07S016JA1R1500:DX07S016JA1R1500: USB-C (USB TYPE-C) USB 2.0 Receptacle Connector 24 (16+8 Dummy) Position Surface Mount, Right Angle; Through Hole; DESCRIPTION: USB-C (USB TYPE-C) USB 2.0 Receptacle Connector 24 (16+8 Dummy) Position Surface Mount, Right Angle; Through Hole; DIGI-KEY_PART_NUMBER: 670-DX07S016JA1R1500CT-ND; MF: JAE Electronics; MP: DX07S016JA1R1500; PACKAGE: None; PURCHASE-URL: https://pricing.snapeda.com/search/part/DX07S016JA1R1500/?ref=eda
J6 = EDCPSU:OLED_LCD
JP1 = 20021521-00010T1LF:20021521-00010T1LF: MINITEK 127 SHROUDED HDR Source: http://portal.fciconnect.com/Comergent//fci/drawing/20021521.pdf; DESCRIPTION: Minitek127®, Shrouded Board to Board Header, Surface Mount, 10 positions, 1.27mm (0.500in) pitch.; DIGI-KEY_PART_NUMBER: 609-4054-ND; MF: AMPHENOL ICC / FCI; MP: 20021521-00010T1LF; PACKAGE: None; PURCHASE-URL: https://pricing.snapeda.com/search/part/20021521-00010T1LF/?ref=eda
K1 = Flex_3mm:FLEX8: WR-FPC 1mm SMT Horiz. Bot. Contact Hinge type WR-FPC 1mm 08 pins Hinge type SMT Horizontal Bottom Contact ;=>Code : Con_FPC_ZIF_1.00_6861xx148922_686108148922 Details see: http://katalog.we-online.de/em/datasheet/6861xx148922.pdf Created 2014-10-08, Karrer Zheng 2014 (C) Wurth Elektronik
L1 = NRS4018T4R7MDGJ:NRS4018T4R7MDGJ: Inductor SMD wirewound 4.7uH; ARROW_PART_NUMBER: NRS4018T4R7MDGJ; ARROW_PRICE-STOCK: https://www.arrow.com/en/products/nrs4018t4r7mdgj/taiyo-yuden; DESCRIPTION: Inductor SMD wirewound 4.7uH; HEIGHT: 1mm; MANUFACTURER_NAME: TAIYO YUDEN; MANUFACTURER_PART_NUMBER: NRS4018T4R7MDGJ; MOUSER_PART_NUMBER: 963-NRS4018T4R7MDGJ; MOUSER_PRICE-STOCK: https://www.mouser.co.uk/ProductDetail/Taiyo-Yuden/NRS4018T4R7MDGJ?qs=PzICbMaShUfBUWy4ytltsA%3D%3D
L2 = EDCPSU - Rev3:L*
L3-L7 = SparkFun:RESISTOR: Resistor
LED1 = SparkFun-LED:LED: LEDs
LS1 = SMT-0540-S-R:SMT-0540-S-R: Speakers & Transducers SMD TRANSDUCER 3VP-P 100MA Source: Datasheet; DESCRIPTION: Speakers & Transducers SMD TRANSDUCER 3VP-P 100MA; HEIGHT: 2mm; MANUFACTURER_NAME: PUI Audio; MANUFACTURER_PART_NUMBER: SMT-0540-S-R; MOUSER_PART_NUMBER: 665-SMT0540SR; MOUSER_PRICE-STOCK: https://www.mouser.co.uk/ProductDetail/PUI-Audio/SMT-0540-S-R?qs=e16JbV5WBEu5VaDVzQP23Q%3D%3D
OP1 = optocoupler:LTV816: OPTO COUPLER Source: LITEON, LTV816.pdf; OC_FARNELL: unknown; OC_NEWARK: unknown
PTC1 = EDCPSU:PTC-: Positive Temperature Coefficient Resistor (PTC)
Q2 Q4 Q5 Q9 = SparkFun-DiscreteSemi:MOSFET-NCHANNEL: Common NMOSFET Parts MFG P/NStore IDProd ID FDD8780TRANS-09984 SI7820DNTRANS-11055 FDS6630AIC-08089 2N7002PWTRANS-11151 FQP30N06L COM-10213TRANS-10060 BSS123LT1GTRANS-08345 BSS138TRANS-00830 BS170 2N7000; PROD_ID: TRANS-11151
R1-R11 R13-R63 R65 R66 R99 RSENSE = SparkFun-Resistors:RESISTOR: Generic Resistor Package
R12 = eagle-ltspice:R: RESISTOR, European symbol; SPICEMODEL: NONE; SPICEPREFIX: R
S1 = SparkFun-Electromechanical:ROTARTY_ENCODER: Simple no LED rotary encoder Example: COM-09117
S2 = EDCPSU - Rev2:TAC_SWITCH: Momentary Switch Button commonly used for reset or general input. Spark Fun Electronics SKU : COM-00097 SMT- SWCH-08247
U1 = RP2040TR7:RP2040TR7: ARM MCU, RP2040 Series Microcontrollers, ARM Cortex-M0+, 32 bit, 133 MHz, 16 MB, 56 Pins Source: Datasheet; DESCRIPTION: ARM MCU, RP2040 Series Microcontrollers, ARM Cortex-M0+, 32 bit, 133 MHz, 16 MB, 56 Pins; HEIGHT: 0.9mm; MANUFACTURER_NAME: RASPBERRY-PI; MANUFACTURER_PART_NUMBER: RP2040TR7
U2 = SparkFun-IC-Conversion:MCP4725: MCP4725 DAC Microchip 12-bit I2C DAC, SOT23-6 Datasheet SparkFun Products SparkFun I2C DAC Breakout - MCP4725 (BOB-12918); PROD_ID: IC-08886
U3 U6 = 74xx-eu:74*14: Hex schmitt trigger INVERTER
U4 = MAX9938:MAX9938FEUK+T; DESCRIPTION: Precision Current-Sense Amplifier; MPN: MAX9938FEUK+T; OC_FARNELL: -; OC_NEWARK: 01N6733; PACKAGE: SOT-23-5; SUPPLIER: Maxim
U5 = W25Q64JVSSIQ:W25Q64JVSSIQ: 64M-bit Serial Flash Memory with uniform 4KB sectors and Dual/Quad SPI Source: Datasheet; ARROW_PART_NUMBER: W25Q64JVSSIQ; ARROW_PRICE-STOCK: https://www.arrow.com/en/products/w25q64jvssiq/winbond-electronics?region=nac; DESCRIPTION: 64M-bit Serial Flash Memory with uniform 4KB sectors and Dual/Quad SPI; HEIGHT: 2.16mm; MANUFACTURER_NAME: Winbond; MANUFACTURER_PART_NUMBER: W25Q64JVSSIQ; MOUSER_PART_NUMBER: 454-W25Q64JVSSIQ; MOUSER_PRICE-STOCK: https://www.mouser.co.uk/ProductDetail/Winbond/W25Q64JVSSIQ?qs=qSfuJ%252Bfl%2Fd4DecxlHDmB8w%3D%3D
U7 = EDCPSU - Rev2:TPIC2810D
U8 = LM4040C30FTA:LM4040C30FTA: Diodes Inc LM4040C30FTA, Shunt Precision Voltage Reference 2.5V, 0.5%, 3-Pin SOT-23 Source: Datasheet; ARROW_PART_NUMBER: LM4040C30FTA; ARROW_PRICE-STOCK: https://www.arrow.com/en/products/lm4040c30fta/diodes-incorporated?region=nac; DESCRIPTION: Diodes Inc LM4040C30FTA, Shunt Precision Voltage Reference 2.5V, 0.5%, 3-Pin SOT-23; HEIGHT: 1.2mm; MANUFACTURER_NAME: Diodes Inc.; MANUFACTURER_PART_NUMBER: LM4040C30FTA; MOUSER_PART_NUMBER: 621-LM4040C30FTA; MOUSER_PRICE-STOCK: https://www.mouser.co.uk/ProductDetail/Diodes-Incorporated/LM4040C30FTA?qs=oUsD4qhOtFxJawR8QeoshQ%3D%3D
U9 = MAX9064:MAX9064EUK+T; COPYRIGHT: Copyright (C) 2022 Ultra Librarian. All rights reserved.; DIGI-KEY_PART_NUMBER_1: MAX9064EUK+TCT-ND; DIGI-KEY_PART_NUMBER_2: MAX9064EUK+TDKR-ND; DIGI-KEY_PART_NUMBER_3: MAX9064EUK+TTR-ND; MANUFACTURER_PART_NUMBER: MAX9064EUK+T; MFR_NAME: Maxim Integrated Products
U10 = IP2721:IP2721: TYPEC/PD2.0/PD3.0 Physical Layer IC for USB TYPEC input Interfaces Working voltage: 3V~25V Package: TSSOP16 Source: Datasheet; DESCRIPTION: TYPEC/PD2.0/PD3.0 Physical Layer IC for USB TYPEC input Interfaces Working voltage: 3V~25V Package: TSSOP16; HEIGHT: 1.2mm; MANUFACTURER_NAME: INJOINIC; MANUFACTURER_PART_NUMBER: IP2721
U11 = AP63201WU-7:AP63201WU-7: Switching Voltage Regulators DCDC Conv HV Buck TSOT26 T&R 3K Source: Datasheet; ARROW_PART_NUMBER: AP63201WU-7; ARROW_PRICE-STOCK: https://www.arrow.com/en/products/ap63201wu-7/diodes-incorporated?region=nac; DESCRIPTION: Switching Voltage Regulators DCDC Conv HV Buck TSOT26 T&R 3K; HEIGHT: 1mm; MANUFACTURER_NAME: Diodes Inc.; MANUFACTURER_PART_NUMBER: AP63201WU-7; MOUSER_PART_NUMBER: 621-AP63201WU-7; MOUSER_PRICE-STOCK: https://www.mouser.co.uk/ProductDetail/Diodes-Incorporated/AP63201WU-7?qs=u16ybLDytRaVD%252BU3eG30NA%3D%3D
U12 = AP64501SP-13:AP64501SP-13: Conv DC-DC 3.8V to 40V Synchronous Step Down Single-Out 0.8V to 39V 5A 8-Pin SO EP T/R Source: Datasheet; ARROW_PART_NUMBER: AP64501SP-13; ARROW_PRICE-STOCK: https://www.arrow.com/en/products/ap64501sp-13/diodes-incorporated?region=nac; DESCRIPTION: Conv DC-DC 3.8V to 40V Synchronous Step Down Single-Out 0.8V to 39V 5A 8-Pin SO EP T/R; HEIGHT: 1.63mm; MANUFACTURER_NAME: Diodes Inc.; MANUFACTURER_PART_NUMBER: AP64501SP-13; MOUSER_PART_NUMBER: 621-AP64501SP-13; MOUSER_PRICE-STOCK: https://www.mouser.co.uk/ProductDetail/Diodes-Incorporated/AP64501SP-13?qs=P1JMDcb91o7FS0GU%252BW7TIQ%3D%3D
USB_D+ USB_D- = SparkFun-Jumpers:JUMPER-SMT_2_NO: Normally open jumper
X1 = ABM3C-12.000MHZ-D4Y-T:ABM3C-12.000MHZ-D4Y-T: Abracon 12MHz Crystal +/-30ppm 4-SMD, No Lead 5 x 3 x 1.3mm Source: Datasheet; ARROW_PART_NUMBER: ABM3C-12.000MHZ-D4Y-T; ARROW_PRICE-STOCK: https://www.arrow.com/en/products/abm3c-12.000mhz-d4y-t/abracon?region=nac; DESCRIPTION: Abracon 12MHz Crystal +/-30ppm 4-SMD, No Lead 5 x 3 x 1.3mm; HEIGHT: 1mm; MANUFACTURER_NAME: ABRACON; MANUFACTURER_PART_NUMBER: ABM3C-12.000MHZ-D4Y-T; MOUSER_PART_NUMBER: 815-ABM3C-12-D4YT; MOUSER_PRICE-STOCK: https://www.mouser.co.uk/ProductDetail/ABRACON/ABM3C-12.000MHZ-D4Y-T?qs=hxOQwdLlgeqaOp0z0XDuIQ%3D%3D

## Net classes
1 vcc: width 0.254 mm

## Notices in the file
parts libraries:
SparkFun-Electromechanical: Licensing: Creative Commons ShareAlike 4.0 International - https://creativecommons.org/licenses/by-sa/4.0
SparkFun-DiscreteSemi: Licensing: CC v3.0 Share-Alike You are welcome to use this library for commercial purposes.
